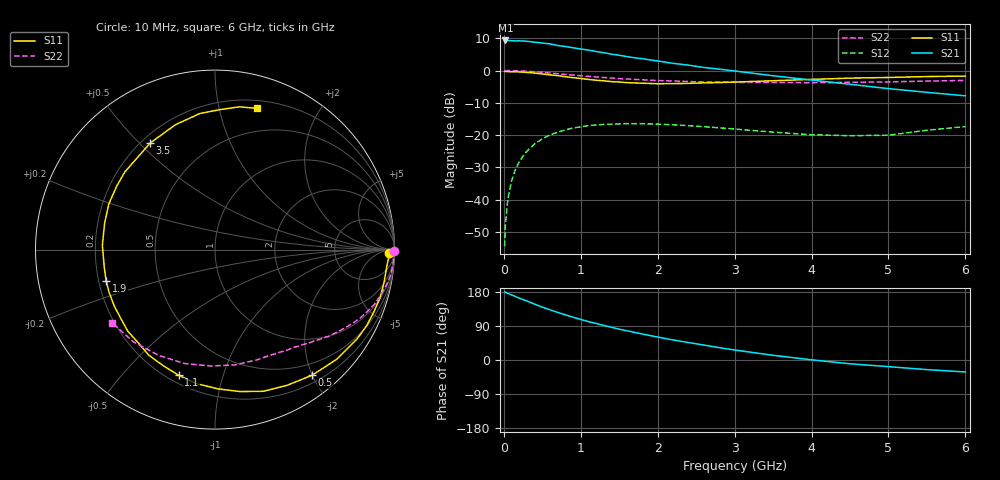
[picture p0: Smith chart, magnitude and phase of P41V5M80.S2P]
! SIEMENS Small Signal Semiconductors
! BFP182
! Si NPN RF Bipolar Junction Transistor in SOT143
! VCE = 1.5 V  IC = 0.8 mA
! Common Emitter S-Parameters:  March  1996
# GHz  S  MA  R  50
!  f  S11  S21  S12  S22
! GHz  MAG  ANG  MAG  ANG  MAG  ANG  MAG  ANG
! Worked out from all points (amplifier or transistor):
!   36 points, 10 MHz to 6 GHz, reference 50 ohm
!   highest |S21| = 9.3 dB at 20 MHz (marker M1)
!   |S21| within 3 dB of that: start of sweep to 1.104 GHz
!   unconditionally stable (mu >= 1): 2.719 GHz to end of sweep
!   at 250 MHz: K = 0.10, MSG = 17.8 dB, |S12| = -26.5 dB
!   at 1.4 GHz: K = 0.52, MSG = 10.8 dB, |S12| = -16.6 dB
!   at 6 GHz: K = 1.17, MAG = 2.3 dB, |S12| = -17.4 dB
!   S11 on the Smith chart (normalised r, x): 10 MHz: 49, -27; 500 MHz: 0.31, -2.00; 1.1 GHz: 0.24, -0.72; 1.9 GHz: 0.23, -0.13; 3.5 GHz: 0.23, +0.54; 6 GHz: 0.27, +1.31
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0.01  0.9691 -1.0  2.917 179.7  0.0019 84.9  0.9987 -0.4
0.02  0.9702 -2.1  2.927 179.0  0.004 91.5  0.9962 -0.8
0.05  0.962 -5.4  2.916 175.9  0.0098 88.5  0.9981 -2.0
0.1  0.9595 -10.7  2.904 171.8  0.0194 83.0  0.9959 -4.0
0.15  0.9582 -16.3  2.882 167.7  0.029 79.9  0.9922 -6.0
0.3  0.9355 -31.9  2.841 155.8  0.0564 70.0  0.9746 -11.9
0.4  0.9131 -42.0  2.754 147.3  0.0729 63.4  0.9572 -15.6
0.5  0.8848 -52.3  2.667 139.5  0.0874 57.2  0.9385 -19.0
0.6  0.8567 -61.8  2.591 132.5  0.1005 51.6  0.915 -22.3
0.8  0.8029 -80.1  2.357 119.1  0.1202 41.2  0.8715 -28.0
1.1  0.7287 -106.2  2.076 101.3  0.1399 28.4  0.8131 -35.0
1.3  0.6943 -122.1  1.887 91.2  0.1466 20.9  0.78 -39.1
1.5  0.6654 -136.9  1.726 81.4  0.1488 14.6  0.7507 -42.7
1.9  0.6309 -164.1  1.463 64.6  0.1489 4.8  0.7093 -49.5
2.2  0.6279 177.9  1.293 52.8  0.1445 -1.1  0.6893 -54.4
2.8  0.6518 147.2  1.052 32.6  0.1297 -8.6  0.6598 -65.2
3.5  0.6949 121.3  0.831 12.4  0.1112 -11.1  0.652 -80.1
4  0.7299 107.6  0.712 0.5  0.1012 -6.7  0.6491 -92.2
4.5  0.7631 96.3  0.613 -10.0  0.0979 -1.1  0.6571 -105.1
5  0.7814 87.6  0.525 -17.5  0.0996 8.7  0.6678 -118.2
5.5  0.8069 80.3  0.46 -25.4  0.1189 12.2  0.6866 -131.8
6  0.8212 73.3  0.406 -31.6  0.1355 12.0  0.7035 -144.7
